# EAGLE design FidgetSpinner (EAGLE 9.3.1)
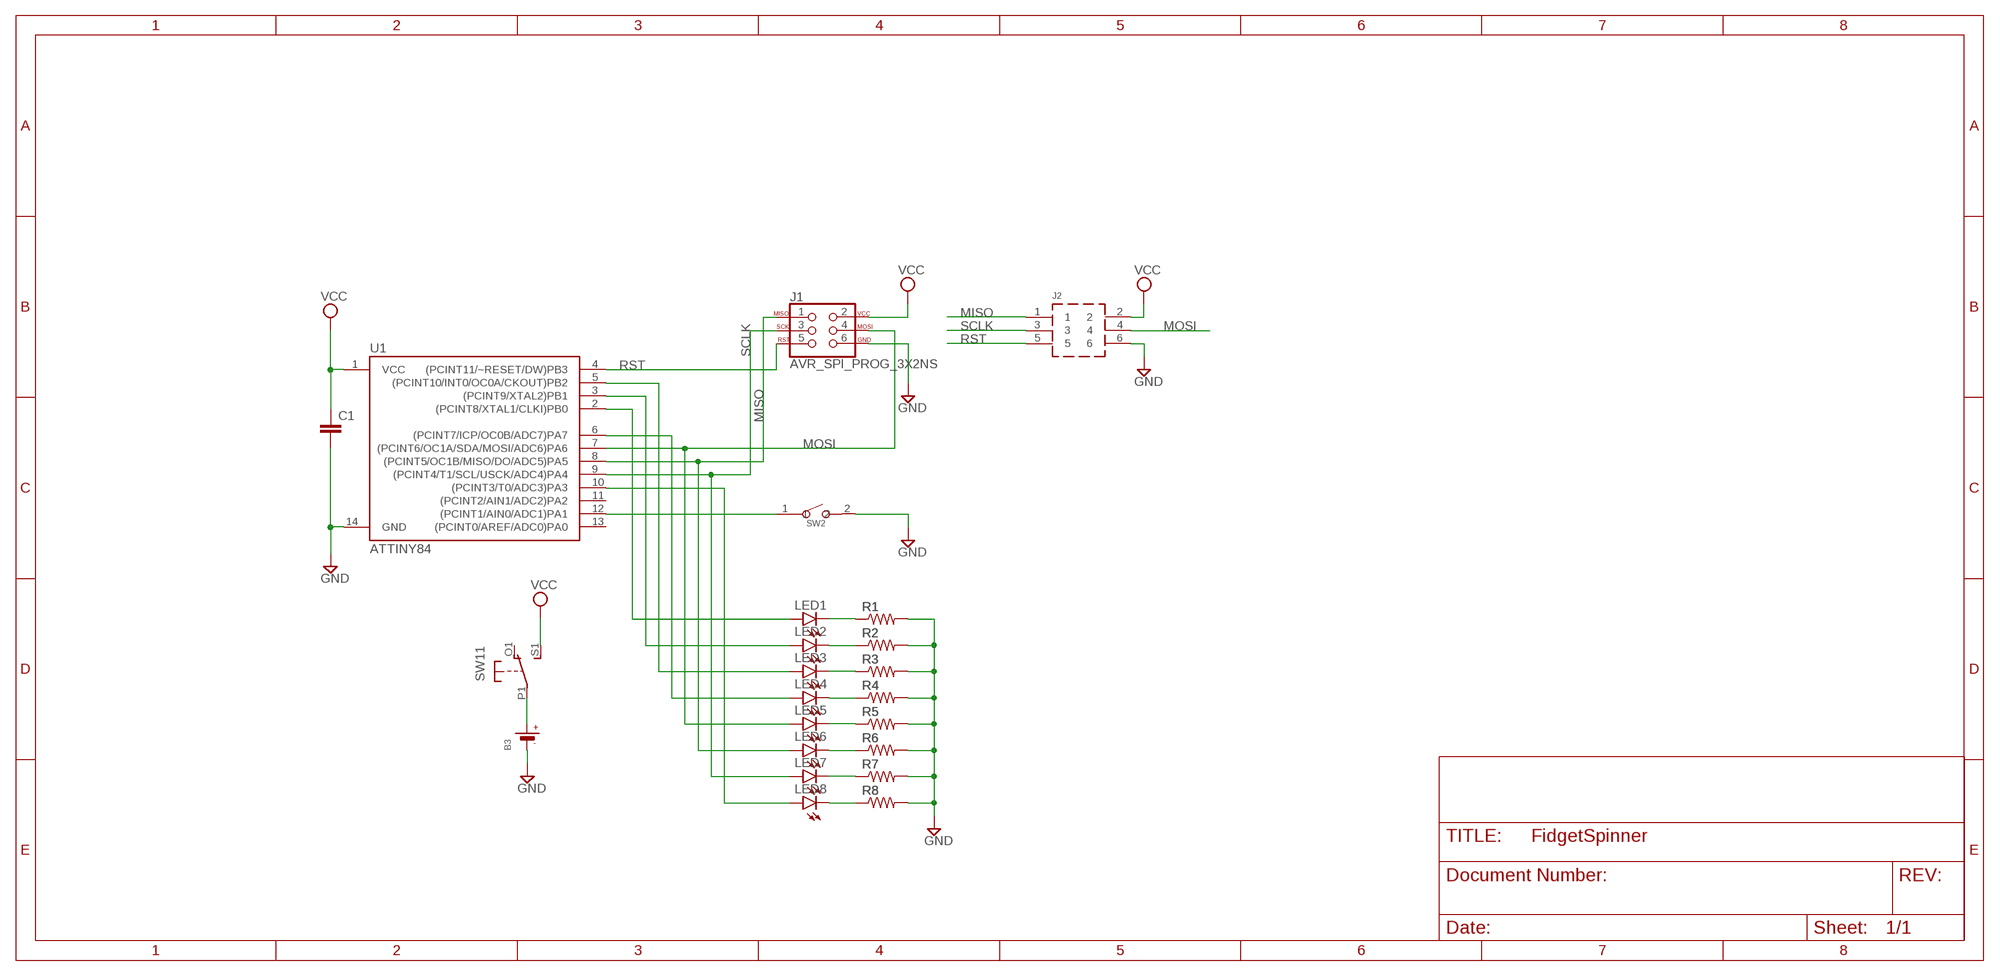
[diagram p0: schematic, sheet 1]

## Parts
B3  BATTERYCR2032_BAT-HLD-001  [CR2032_SMT_BAT-HLD-001]
C1  CAPC0805  [C0805]
J1  AVR_SPI_PROG_3X2NS  [2X3-NS]
J2  610106249121  [RA-SMT-HDR-2X3]
LED1  LEDCHIP-LED0805  [CHIP-LED0805]
LED2  LEDCHIP-LED0805  [CHIP-LED0805]
LED3  LEDCHIP-LED0805  [CHIP-LED0805]
LED4  LEDCHIP-LED0805  [CHIP-LED0805]
LED5  LEDCHIP-LED0805  [CHIP-LED0805]
LED6  LEDCHIP-LED0805  [CHIP-LED0805]
LED7  LEDCHIP-LED0805  [CHIP-LED0805]
LED8  LEDCHIP-LED0805  [CHIP-LED0805]
R1  RESISTORR0805  [R0805]
R2  RESISTORR0805  [R0805]
R3  RESISTORR0805  [R0805]
R4  RESISTORR0805  [R0805]
R5  RESISTORR0805  [R0805]
R6  RESISTORR0805  [R0805]
R7  RESISTORR0805  [R0805]
R8  RESISTORR0805  [R0805]
SW1  DPDT-EG1390  [EG1390]
SW2  B3U-1000P-2P-SMD  SMD-BUTTON(2P-3.0X2.5X1.2+0.4MM)-B3U-1000P-2P-SMD  [SW2-2.6-3.0X2.5X1.2+0.4MM]
U1  ATTINY84  [SO14]

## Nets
GND: B3.- C1.2 J1.6 J2.6 R1.2 R2.2 R3.2 R4.2 R5.2 R6.2 R7.2 R8.2 SW2.2 U1.14(GND)
MISO: J1.1 J2.1 LED6.A U1.8((PCINT5/OC1B/MISO/DO/ADC5)PA5)
MOSI: J1.4 J2.4 LED5.A U1.7((PCINT6/OC1A/SDA/MOSI/ADC6)PA6)
N$3: LED1.C R1.1
N$6: LED2.C R2.1
N$7: LED3.C R3.1
N$8: LED4.C R4.1
N$9: LED5.C R5.1
N$10: LED6.C R6.1
N$11: LED7.C R7.1
N$12: LED8.C R8.1
N$13: LED1.A U1.2((PCINT8/XTAL1/CLKI)PB0)
N$14: LED2.A U1.3((PCINT9/XTAL2)PB1)
N$15: LED3.A U1.5((PCINT10/INT0/OC0A/CKOUT)PB2)
N$16: LED4.A U1.6((PCINT7/ICP/OC0B/ADC7)PA7)
N$17: LED8.A U1.10((PCINT3/T0/ADC3)PA3)
N$19: B3.+$1(+) B3.+$2(+) SW1.P1(1:P)
N$23: SW2.1 U1.12((PCINT1/AIN0/ADC1)PA1)
RST: J1.5 J2.5 U1.4((PCINT11/~RESET/DW)PB3)
SCLK: J1.3 J2.3 LED7.A U1.9((PCINT4/T1/SCL/USCK/ADC4)PA4)
VCC: C1.1 J1.2 J2.2 SW1.S1(1:S) U1.1(VCC)
Unconnected: SW1.O1(1:O) SW1.O2(2:O) SW1.P2(2:P) SW1.S2(2:S) U1.11((PCINT2/AIN1/ADC2)PA2) U1.13((PCINT0/AREF/ADC0)PA0)

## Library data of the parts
B3 = microbuilder:BATTERY: CR1220 SMT - Digikey: 3001K-ND
C1 = LED_Driver:CAP: Capacitor
J1 = SparkFun-Connectors:AVR_SPI_PROG_3X2: AVR ISP 6 Pin This is the reduced ISP connector for AVR programming. Common on Arduino. This footprint will take up less PCB space and can be used with a 10-pin to 6-pin adapter such as SKU: BOB-08508 **Special note about "TEST_POINT" package. The stop mask is on the top side, so if you want your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
J2 = RA-SMT-HDR-2x3:610106249121
LED1-LED8 = led:LED: LED
R1-R8 = LED_Driver:RESISTOR: Resistor
SW1 = adafruit:DPDT
SW2 = Seeed-Switch:SMD-BUTTON(2P-3.0X2.5X1.2+0.4MM): 311020047; MPN: B3U-1000P-2P-SMD; SPICEPREFIX: B
U1 = SparkFun-IC-Microcontroller:ATTINY84: Atmel 14-pin 2/4/8kB flash uC Datasheet SparkFun Products Tiny AVR Programmer (PGM-11801) SparkFun Servo Trigger - Continuous Rotation (WIG-13872) SparkFun Servo Trigger (WIG-13118); PROD_ID: IC-11285

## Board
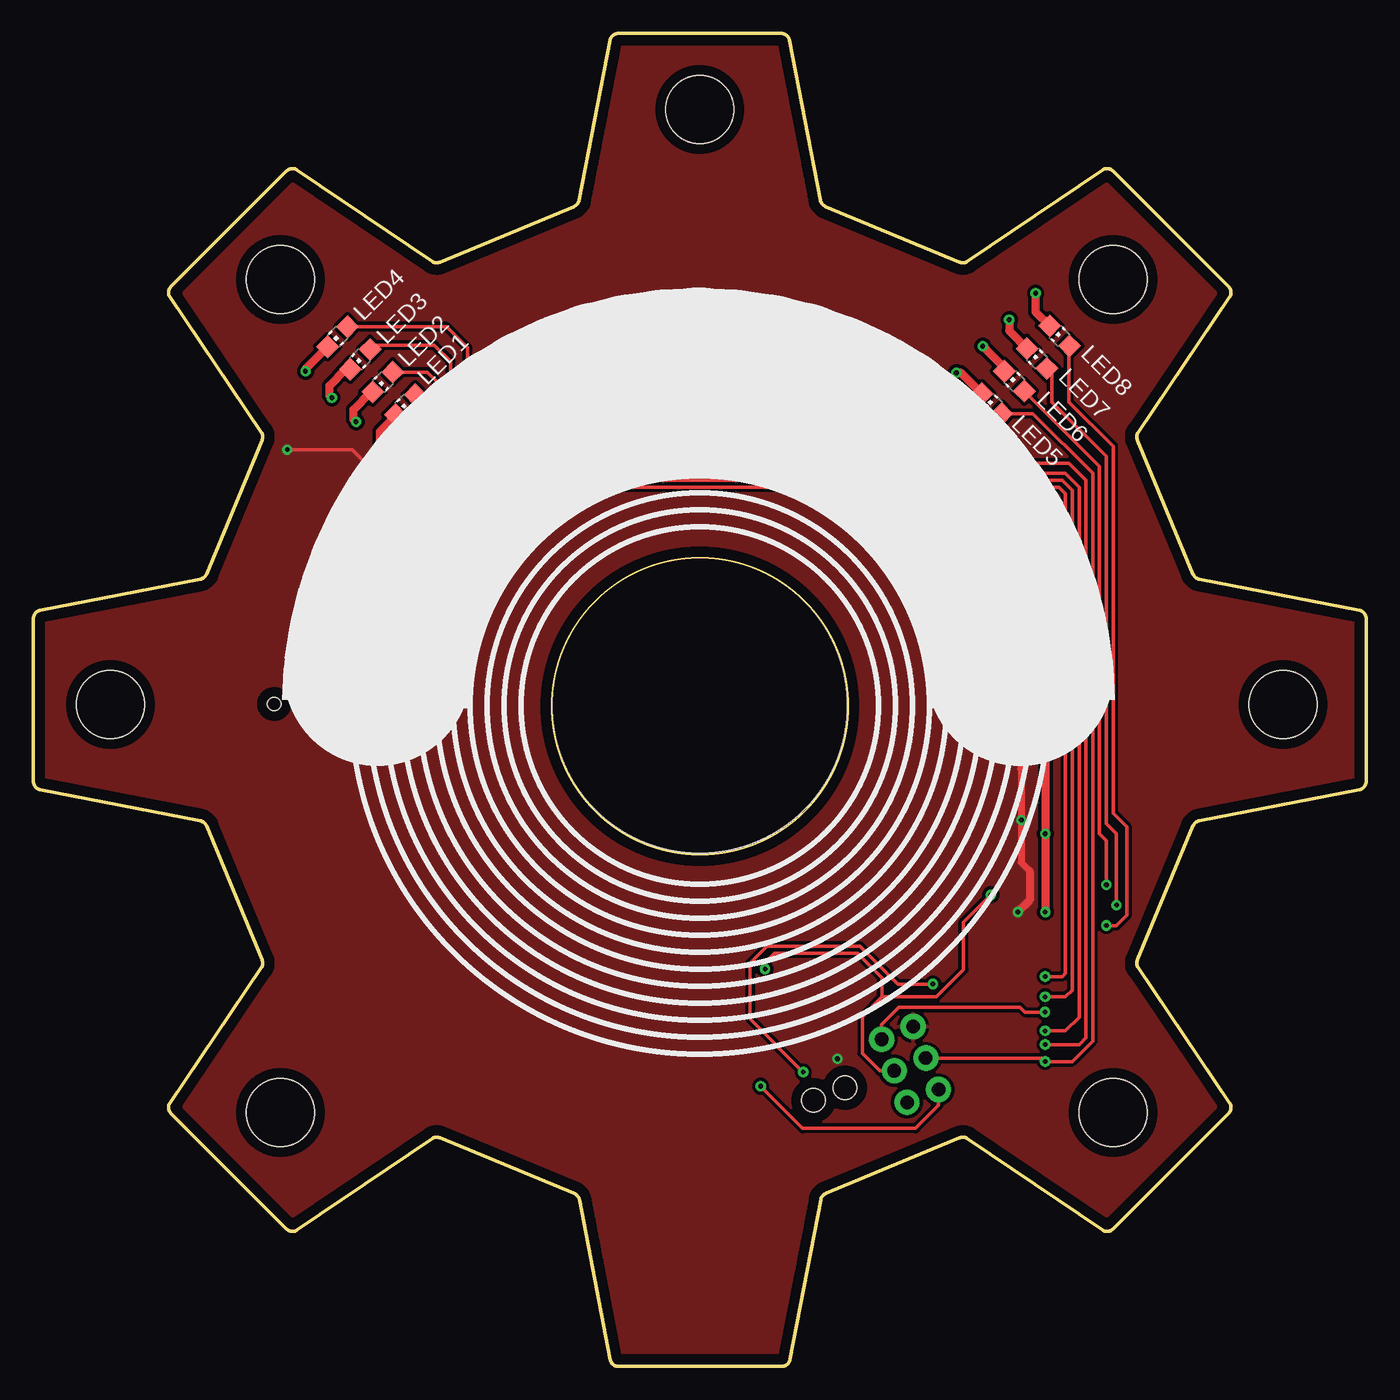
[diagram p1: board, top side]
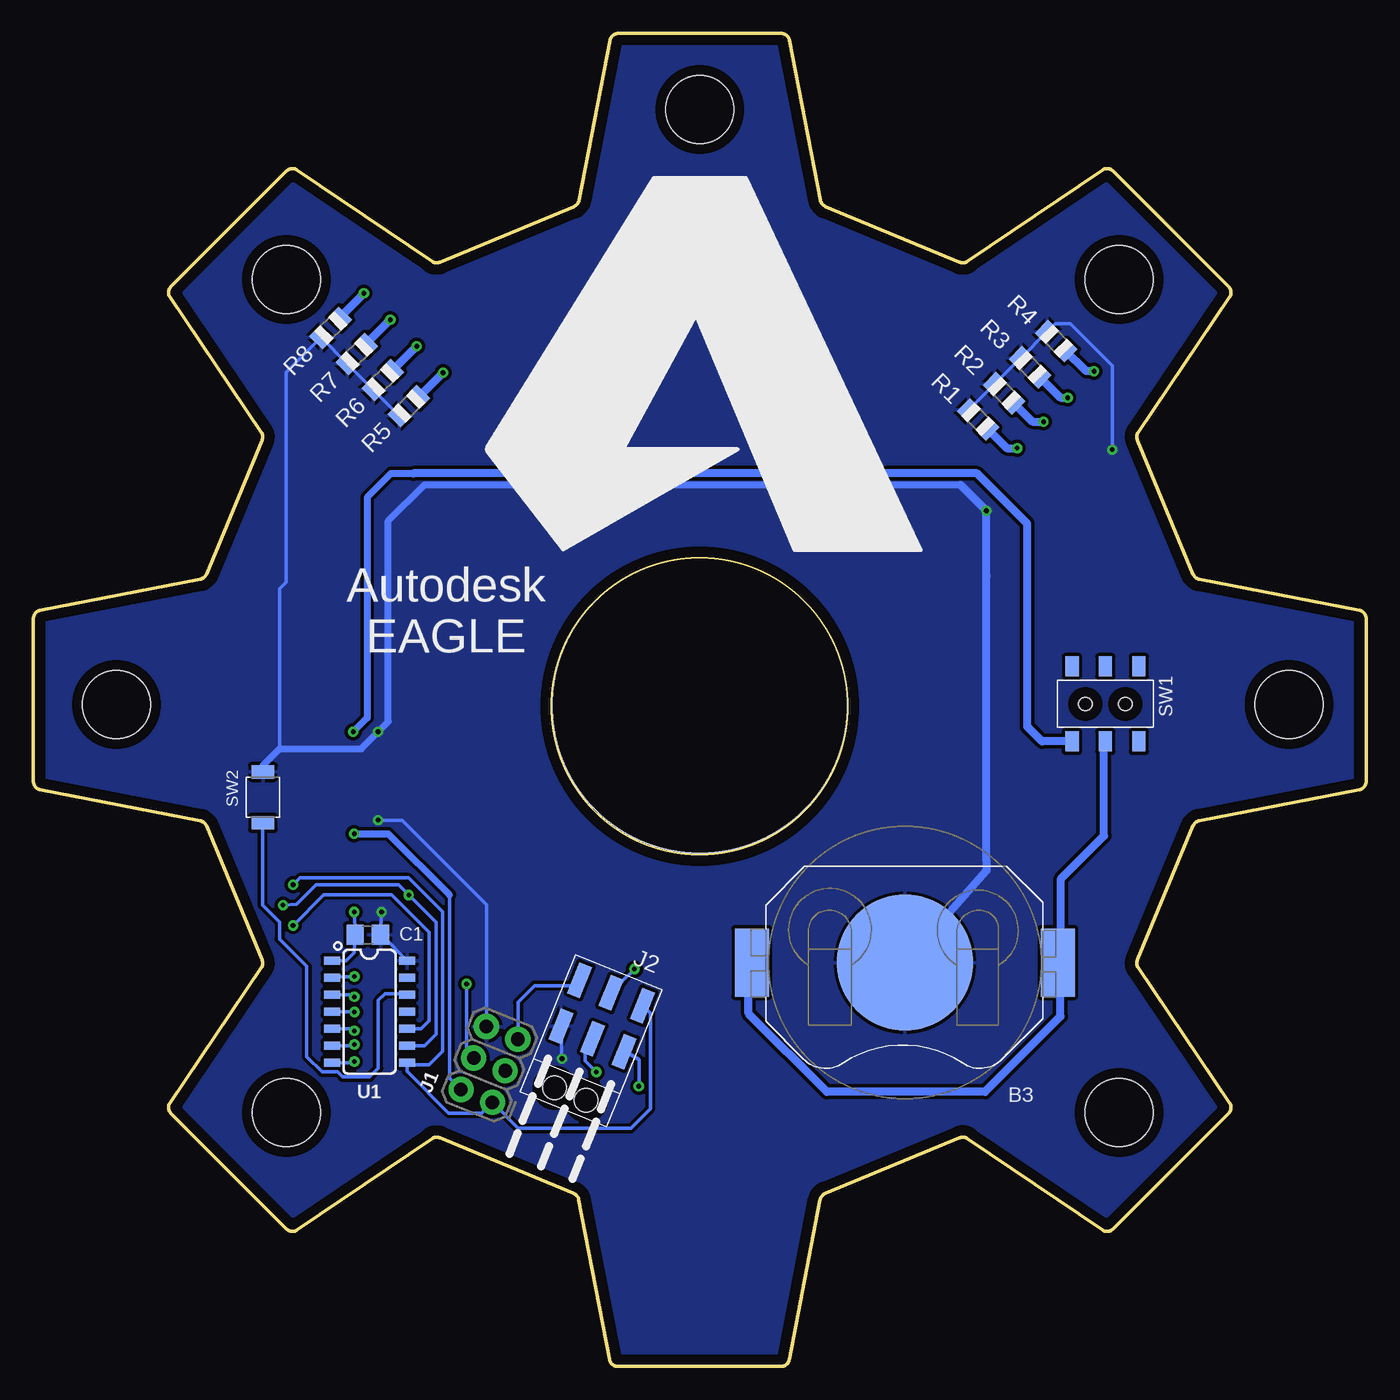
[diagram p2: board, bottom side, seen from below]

Size 99.6 x 99.6 mm. Coordinates in mm from the lower left corner, seen from the top.
Outline: 64 segments
Outline: circle at 49.81,49.33 radius 11.07
Copper layers (1*16): Top 0.035mm / dielectric 1.5mm / Bottom 0.035mm
Design rules "default *": minimum track width 6mil, minimum drill 0.35mm, track to track 10mil, track to pad 10mil, pad to pad 10mil, via to via 10mil, smd to smd 6mil, copper to edge 30mil, drill to drill 6mil, minimum pad ring 10mil, minimum via ring 8mil, stop-mask expansion 4mil, vias tented up to drill 0mil, thermal gap 10mil
Holes 5.08 mm at 18.47,18.97 5.77,49.45 18.47,81.2 49.8,93.9 80.7,81.2 93.4,49.45 80.7,18.97
Holes 22.05 mm at 49.8,49.39

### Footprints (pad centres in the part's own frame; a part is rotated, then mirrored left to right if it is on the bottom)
CR2032_SMT_BAT-HLD-001 = smd 2.54 x 5.08: +$1 -11.43,0; +$2 11.43,0 | smd 10.16 x 10.16: - 0,0
C0805 = smd 1.3 x 1.5: 1 -0.95,0; 2 0.95,0
2X3-NS = drill 1.016 pad 1.88: 1 -2.54,-1.27; 2 -2.54,1.27; 3 0,-1.27; 4 0,1.27; 5 2.54,-1.27; 6 2.54,1.27
RA-SMT-HDR-2X3 = smd 1 x 2.5: 1 0,0; 2 0,3.7; 3 2.54,0; 4 2.54,3.7; 5 5.08,0; 6 5.08,3.7 | hole 1.78: 1.27,8.15; 3.81,8.15
CHIP-LED0805 = smd 1.2 x 1.2: A 0,-1.05; C 0,1.05
R0805 = smd 1.1 x 1.4: 1 -1,0; 2 1,0
EG1390 = smd 1 x 1.5: O1 -2.5,2.8; O2 -2.5,-2.8; P1 0,2.8; P2 0,-2.8; S1 2.5,2.8; S2 2.5,-2.8 | hole 1: 1.5,0; -1.5,0
SW2-2.6-3.0X2.5X1.2+0.4MM = smd 1 x 1.7: 1 -1.9,0; 2 1.9,0
SO14 = smd 0.6 x 1.2: 1 -3.175,-2.8; 2 -1.905,-2.8; 3 -0.635,-2.8; 4 0.635,-2.8; 5 1.905,-2.8; 6 3.175,-2.8; 7 4.445,-2.8; 8 4.445,2.8; 9 3.175,2.8; 10 1.905,2.8; 11 0.635,2.8; 12 -0.635,2.8; 13 -1.905,2.8; 14 -3.175,2.8

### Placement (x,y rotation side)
B3  34.47,30.18 0 bottom
C1  74.61,32.24 0 bottom
J1  65.52,22.57 68 bottom
J2  54.07,26.96 158 bottom
LED1  27.8,71.87 135 top
LED2  26.11,73.56 135 top
LED3  24.42,75.25 135 top
LED4  22.73,76.94 135 top
LED5  71.63,71.93 45 top
LED6  73.32,73.62 45 top
LED7  75.01,75.31 45 top
LED8  76.7,77 45 top
R1  29,70.77 135 bottom
R2  27.06,72.71 135 bottom
R3  25.11,74.66 135 bottom
R4  23.16,76.6 135 bottom
R5  71.55,71.75 225 bottom
R6  73.5,73.7 225 bottom
R7  75.44,75.64 225 bottom
R8  77.39,77.59 225 bottom
SW1  19.48,49.51 180 bottom
SW2  82.45,42.52 90 bottom
U1  74.48,27.14 270 bottom

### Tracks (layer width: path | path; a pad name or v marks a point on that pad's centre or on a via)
GND  (via drill 0.35)
  Top 0.254: v18.98,68.5 23.8,68.5 v28.37,63.93
  Top 0.508: 73.84,44.63 v73.84,40.82 73.84,37.64 74.47,37.01
  Top 0.61: 74.47,37.01 74.47,34.85 v73.59,33.96 | v73.84,47.42 73.84,44.63
  Bottom 0.254: U1.14 73.6,32.24 C1.2 73.61,33.93 v73.59,33.96 | R5.2 R6.2 R7.2 R8.2 80.7,74.28 80.7,58.6 81.21,58.09 81.21,46.15 | R1.2 27.73,73.38 R2.2 25.78,75.33 | 25.78,75.33 R3.2 | 25.78,75.33 R4.2 23.21,77.9 22.1,77.9 18.98,74.78 v18.98,68.5 | J1.6 65.75,34.51 72.06,40.82 v73.84,40.82 | v60.1,22.99 60.15,22.99 60.15,24.38 60.16,24.36 J2.6
  Bottom 0.508: 30.3,65.86 70.39,65.86 73.08,63.17 73.08,48.18 v73.84,47.42 75.11,46.15 81.21,46.15 82.45,44.91 SW2.2
  Bottom 0.61: 30.3,65.86 v28.37,63.93 28.37,59.06 28.37,37.76 28.37,37.06 B3.-
  pour Bottom: 30.39,17.08 40.41,12.94 arc-57 40.8,12.47 43.1,0.52 arc79 43.74,0 55.91,0 arc79 56.54,0.52 58.85,12.47 arc-57 59.23,12.94 69.22,17.08 arc-57 69.82,17.02 79.9,10.2 arc79 80.71,10.28 89.32,18.89 arc79 89.4,19.7 82.58,29.78 arc-57 82.52,30.38 86.67,40.39 arc-57 87.14,40.77 99.08,43.08 arc79 99.6,43.71 99.6,55.88 arc79 99.08,56.51 87.14,58.82 arc-57 86.67,59.2 82.52,69.21 arc-57 82.58,69.82 89.4,79.89 arc79 89.32,80.71 80.71,89.32 arc79 79.9,89.39 69.82,82.58 arc-57 69.22,82.52 59.21,86.66 arc-57 58.83,87.13 56.52,99.08 arc79 55.89,99.6 43.71,99.6 arc79 43.08,99.08 40.78,87.13 arc-57 40.39,86.66 30.39,82.52 arc-57 29.78,82.58 19.71,89.39 arc79 18.89,89.32 10.28,80.71 arc79 10.2,79.89 17.02,69.82 arc-57 17.08,69.21 12.94,59.2 arc-57 12.47,58.82 0.52,56.51 arc79 0,55.88 0,43.71 arc79 0.52,43.08 12.47,40.77 arc-57 12.94,40.39 17.08,30.38 arc-57 17.02,29.78 10.2,19.7 arc79 10.28,18.89 18.89,10.28 arc79 19.71,10.2 29.78,17.02 arc-57
  pour Top: 19.71,10.2 29.78,17.02 arc-57 30.39,17.08 40.41,12.94 arc-57 40.8,12.47 43.1,0.52 arc79 43.74,0 55.91,0 arc79 56.54,0.52 58.85,12.47 arc-57 59.23,12.94 69.22,17.08 arc-57 69.82,17.02 79.9,10.2 arc79 80.71,10.28 89.32,18.89 arc79 89.4,19.7 82.58,29.78 arc-57 82.52,30.38 86.67,40.39 arc-57 87.14,40.77 99.08,43.08 arc79 99.6,43.71 99.6,55.88 arc79 99.08,56.51 87.14,58.82 arc-57 86.67,59.2 82.52,69.21 arc-57 82.58,69.82 89.4,79.89 arc79 89.32,80.71 80.71,89.32 arc79 79.9,89.39 69.82,82.58 arc-57 69.22,82.52 59.21,86.66 arc-57 58.83,87.13 56.52,99.08 arc79 55.89,99.6 43.71,99.6 arc79 43.08,99.08 40.78,87.13 arc-57 40.39,86.66 30.39,82.52 arc-57 29.78,82.58 19.71,89.39 arc79 18.89,89.32 10.28,80.71 arc79 10.2,79.89 17.02,69.82 arc-57 17.08,69.21 12.94,59.2 arc-57 12.47,58.82 0.52,56.51 arc79 0,55.88 0,43.71 arc79 0.52,43.08 12.47,40.77 arc-57 12.94,40.39 17.08,30.38 arc-57 17.02,29.78 10.2,19.7 arc79 10.28,18.89 18.89,10.28 arc79
MISO  (via drill 0.35)
  Top 0.254: v80.19,35.99 80.19,39.29 79.68,39.8 79.68,67.26 LED6.A
  Bottom 0.254: v80.19,35.99 79.68,36.5 71.55,36.5 69.01,33.96 69.01,23.55 70.03,22.53 71.51,22.53 U1.8 71.68,22.04 68.56,18.92 66.11,18.92 J1.1 63.37,17.8 54.95,17.8 53.48,19.26 53.48,26.38 J2.1
MOSI  (via drill 0.35)
  Top 0.254: v75.62,22.78 75.36,23.04 J1.4 75.61,23.04 75.87,22.78 77.65,22.78 79.17,24.31 79.17,66.73 74.71,71.19 LED5.A | v67.24,28.58 64.6,28.58 61.78,31.4 54.81,31.4 53.54,30.13 53.54,26.06 53.6,25.93 v57.53,22
  Bottom 0.254: v75.62,22.78 75.7,22.7 U1.7 | J1.4 67.24,23.58 v67.24,28.58 | J2.4 58.37,23.92 58.37,22.84 v57.53,22
N$3  (via drill 0.35)
  Top 0.61: v26.08,68.61 25.9,68.79 25.9,69.87 27.06,71.03 LED1.C
  Bottom 0.61: R1.1 26.85,68.61 v26.08,68.61
N$6  (via drill 0.35)
  Top 0.61: v24.1,70.59 23.92,70.77 23.92,71.49 25.25,72.81 LED2.C
  Bottom 0.61: R2.1 24.93,70.59 v24.1,70.59
N$7  (via drill 0.35)
  Top 0.61: v22.31,72.39 22.13,72.57 22.13,73.28 23.35,74.5 LED3.C
  Bottom 0.61: R3.1 22.84,72.39 v22.31,72.39
N$8  (via drill 0.35)
  Top 0.61: LED4.C 20.33,74.54 v20.33,74.36
  Bottom 0.61: v20.33,74.36 20.92,74.36 R4.1
N$9  (via drill 0.35)
  Top 0.61: v68.98,74.25 69.3,74.25 LED5.C
  Bottom 0.61: R5.1 70.81,72.42 v68.98,74.25
N$10  (via drill 0.35)
  Top 0.61: LED6.C 72.58,74.61 v70.96,76.23
  Bottom 0.61: v70.96,76.23 v70.97,76.23 R6.1
N$11  (via drill 0.35)
  Top 0.61: v72.93,78.21 72.93,77.39 LED7.C
  Bottom 0.61: R7.1 74.77,76.36 v72.93,78.21
N$12  (via drill 0.35)
  Top 0.61: v74.91,80.18 74.91,78.79 LED8.C
  Bottom 0.61: R8.1 76.72,78.37 v74.91,80.18
N$13  (via drill 0.35)
  Top 0.254: v75.62,29.13 76.89,29.13 77.14,29.39 77.14,65.2 76.63,65.71 31.42,65.71 28.54,68.59 LED1.A
  Bottom 0.254: v75.62,29.13 77.19,29.13 U1.2
N$14  (via drill 0.35)
  Top 0.254: v75.62,27.61 77.14,27.61 77.65,28.12 77.65,65.46 76.89,66.22 33.2,66.22 30.15,69.27 30.15,73.58 29.44,74.3 LED2.A
  Bottom 0.254: v75.62,27.61 75.79,27.78 U1.3
N$15  (via drill 0.35)
  Top 0.254: LED3.A 25.16,76.32 29.96,76.32 31.17,75.11 31.17,70.03 34.47,66.73 77.14,66.73 78.16,65.71 78.16,26.09 77.14,25.07 v75.62,25.07
  Bottom 0.254: v75.62,25.07 75.79,25.24 U1.5
N$16  (via drill 0.35)
  Top 0.254: LED4.A 23.8,77.68 30.89,77.68 32.44,76.12 32.44,71.04 35.99,67.49 77.4,67.49 78.67,66.22 78.67,24.56 78.16,24.05 v75.62,24.05
  Bottom 0.254: v75.62,24.05 75.7,23.97 U1.6
N$17  (via drill 0.35)
  Top 0.254: LED8.A 77.4,76.21 77.4,72.06 80.7,68.76 80.7,41.33 81.71,40.31 81.71,33.7 80.95,32.94 v80.19,32.94
  Bottom 0.254: U1.10 70.62,25.24 70.03,25.83 70.03,32.44 72.82,35.23 77.9,35.23 v80.19,32.94
N$19
  Bottom 0.61: SW1.P1 19.59,46.6 19.59,39.65 22.84,36.4 22.84,30.76 22.58,30.51 22.91,30.18 | 22.91,30.18 B3.+$2 | 22.91,30.18 22.84,30.1 22.84,26.16 28.48,20.52 40.31,20.52 46.15,26.37 46.15,29.92 B3.+$1
N$23
  Bottom 0.254: U1.12 71.76,27.86 73.33,27.86 73.84,27.36 73.84,22.28 74.47,21.64 76.51,21.64 76.88,22.02 78.04,22.02 79.17,23.16 79.17,29.9 81.21,31.93 81.21,33.2 81.62,33.62 | 81.62,33.62 82.48,34.47 | 82.48,34.47 81.62,33.62 | 82.48,40.59 SW2.1 82.48,40.59 | 82.48,34.47 82.48,40.59
RST  (via drill 0.35)
  Top 0.254: v75.61,26.48 74.09,26.48 73.73,26.85 64.7,26.85 63.4,25.55 J1.5
  Bottom 0.254: U1.4 75.66,26.51 75.65,26.52 v75.61,26.48 | J1.5 63.4,27.21 62.16,28.45 59.33,28.45 59.23,28.41 J2.5
SCLK  (via drill 0.35)
  Top 0.254: v80.95,34.47 80.95,39.8 80.19,40.56 80.19,68 76.13,72.06 76.13,74.19 LED7.A | v71.55,35.23 69.52,33.2 69.52,29.64 67.49,27.61 63.43,27.61 | J1.3 63.27,22.09 61.95,23.41 61.95,26.13 63.43,27.61 | 63.43,27.61 63.43,29.03 61.57,30.89 55.37,30.89 54.69,30.2 v54.69,29.69
  Bottom 0.254: v80.95,34.47 79.92,34.55 78.48,35.99 72.32,35.99 v71.55,35.23 69.52,33.2 69.52,24.82 70.37,23.97 U1.9 | J2.3 55.6,28.74 55.6,28.78 v54.69,29.69
VCC  (via drill 0.35)
  Top 0.254: J1.2 67.65,19.52 65.93,17.8 57.49,17.8 56.14,19.15 v54.36,20.93
  Top 0.61: v75.63,33.95 v75.63,39.8 75.63,47.42 v75.7,47.42
  Bottom 0.254: v75.63,33.95 75.61,33.94 C1.1 75.63,30.91 76.22,30.32 U1.1 | 68.51,35.23 68.51,21.54 J1.2 | J2.2 55.3,23.53 54.38,22.97 54.36,22.93 v54.36,20.93
  Bottom 0.508: 71.2,66.73 72.86,66.73 74.65,64.93 74.65,48.47 v75.7,47.42 | v75.63,39.8 73.08,39.8 68.51,35.23
  Bottom 0.61: SW1.S1 24.23,46.71 25.33,47.8 25.33,62.97 29.08,66.73 71.2,66.73

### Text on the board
bPlace: Autodesk / EAGLE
